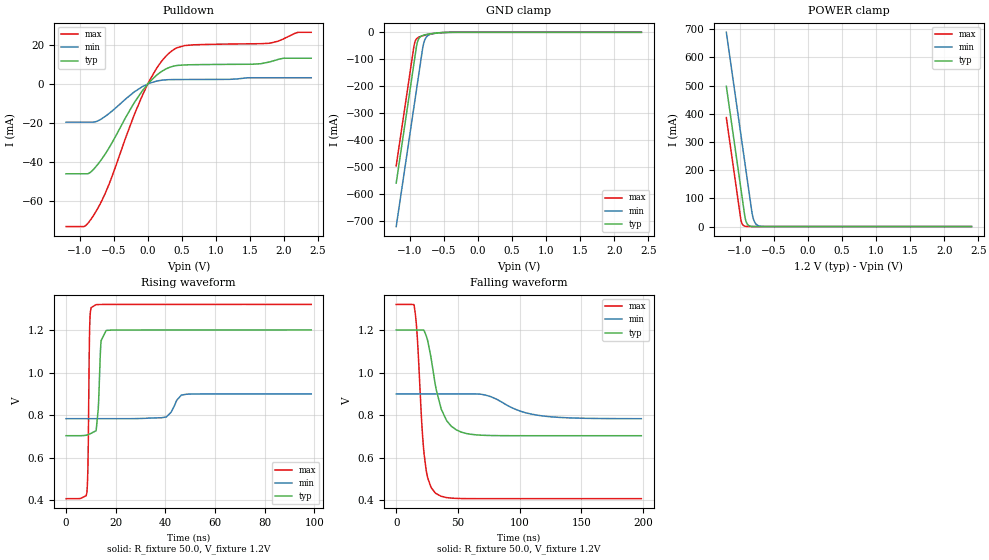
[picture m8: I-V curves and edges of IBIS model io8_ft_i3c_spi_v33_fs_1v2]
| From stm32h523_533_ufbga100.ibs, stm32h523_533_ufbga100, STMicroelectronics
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[Model]   io8_ft_i3c_spi_v33_fs_1v2
Model_type I/O_open_drain
Polarity   Non-Inverting
Enable   Active-Low
| CAP_THRESHOLD on pad IOFT is "UDTCAPC" :
| Rising=20.0% of vddiom   Falling=80.0% of vddiom
| C_comp min and max val. don't necessarily correlate with the min and max pvt
| but are the smallest and greatest pad capacitance found.
| var   typ   min   max
C_comp   3.39520pF  3.36985pF  3.42675pF
|C_comp_pulldown   3.39520pF  3.36985pF  3.42675pF
Vinl = 450.0mV
Vinh = 660.0mV
Vmeas = 600.0mV   | Reference voltage for timing measurements
Cref  = 50.0pF   | Timing specification test load capacitance value
Rref  = 1.0MOhm   | Timing specification test load resistance value
Vref  = 660.0mV   | Timing specification test load voltage
[Model Spec]
| TIME_THRESHOLD on pin ZII2CV11 is "CMOS" :
| Rising=40.0% of vdd   Falling=60.0% of vdd
Vinl 437.80000mV 335.80000mV 479.80000mV
Vinh 728.20000mV 529.20000mV 807.20000mV
| variable   typ   min   max
[Temperature Range] 25.0 125.0 -40.0
| variable   typ   min   max
[Voltage Range] 1.2V 900.0mV 1.32V
| variable   typ   min   max
[POWER Clamp Reference] 1.2V 900.0mV 1.32V
| variable   typ   min   max
[GND Clamp Reference] 0V 0V 0V
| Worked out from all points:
|   slope of the pulldown table from 0 to 0.18 V, typ, clamps not added: 30.6 ohm
|   GND clamp passes 1 mA (typ) near -0.52 V on its own axis
|   POWER clamp passes 1 mA (typ) near -0.84 V on its own axis
|   rising waveform, R_fixture 50.0, V_fixture 1.2V: 20-80 % time 1.11ns typ, 3.39ns min, 533ps max; typ from 0.704 V to 1.2 V
|   falling waveform, R_fixture 50.0, V_fixture 1.2V: 20-80 % time 11.4ns typ, 27.5ns min, 5.82ns max; typ from 1.2 V to 0.704 V
[POWER Clamp]
-1.2V     497.8mA    689.2mA    386.5mA
-990mV    140.8mA    332.2mA    29.53mA
-980mV    123.8mA    315.2mA    17.95mA
-960mV    89.81mA    281.2mA    6.634mA
-930mV    38.81mA    230.2mA    1.49mA
-900mV    12.07mA    179.2mA    334.8uA
-870mV    3.756mA    128.2mA    75.22uA
-820mV    536.4uA    44.98mA    6.246uA
-790mV    166.9uA    18.76mA    1.403uA
-750mV    35.18uA    5.846mA    191.8nA
-590mV    70.09nA    55uA       165.5pA
2.4V      0A         0A         0A
[GND Clamp]
-1.2V     -558.2mA   -719mA     -494.1mA
-940mV    -116.2mA   -277mA     -52.06mA
-930mV    -99.19mA   -260mA     -39.94mA
-900mV    -49.1mA    -209mA     -23.76mA
-880mV    -30.14mA   -175mA     -19.6mA
-850mV    -17.82mA   -124mA     -16.09mA
-810mV    -11.73mA   -56.78mA   -12.91mA
-780mV    -9.444mA   -28.21mA   -10.92mA
-740mV    -7.291mA   -13.16mA   -8.574mA
-640mV    -3.573mA   -4.171mA   -3.954mA
-380mV    -61.75uA   -230.3uA   -20.32uA
2.4V      3.863nA    718.4nA    150.6pA
| variable   typ   min   max
[Pullup Reference] 1.2V 900.0mV 1.32V
| variable   typ   min   max
[Pulldown Reference] 0V 0V 0V
[Pulldown]
-1.2V     -46.17mA   -19.62mA   -73.27mA
-930mV    -46.17mA   -19.62mA   -73.18mA
-770mV    -42.8mA    -19.41mA   -66.04mA
-570mV    -32.88mA   -15.18mA   -51.58mA
-200mV    -9.658mA   -4.083mA   -15.89mA
-80mV     -3.488mA   -1.363mA   -5.887mA
120mV     4.232mA    1.387mA    7.501mA
340mV     8.782mA    2.251mA    16.66mA
540mV     9.805mA    2.305mA    19.74mA
1.79V     11.33mA    3.206mA    20.93mA
2.2V      13.23mA    3.206mA    26.48mA
2.4V      13.23mA    3.206mA    26.56mA
[Ramp]
dV/dt_r 297.79762mV/1.02964ns 69.90051mV/3.06045ns 547.1337mV/532.05683ps
dV/dt_f 297.80511mV/10.9787ns 69.80217mV/27.29122ns 547.13933mV/5.72638ns
R_load = 50.0
| Removed startup time: 0s 0s 0s  .
| Removed end time: 98.75ns.
[Rising Waveform]
R_fixture   = 50.0
V_fixture   = 1.2V
V_fixture_min = 900.0mV
V_fixture_max = 1.32V
0s        703.7mV    783.5mV    408.1mV
8.35ns    706.4mV    783.5mV    435.3mV
8.85ns    708.5mV    783.5mV    589.5mV
9.5ns     711.7mV    783.5mV    1.21V
10.1ns    715.1mV    783.5mV    1.305V
12.1ns    727mV      783.5mV    1.319V
12.95ns   827.9mV    783.5mV    1.319V
14.1ns    1.15V      783.5mV    1.32V
16.15ns   1.198V     783.5mV    1.32V
98.75ns   1.2V       900mV      1.32V
| Removed startup time: 0s 0s 0s  .
| Removed end time: 198.75ns.
[Falling Waveform]
R_fixture   = 50.0
V_fixture   = 1.2V
V_fixture_min = 900.0mV
V_fixture_max = 1.32V
0s        1.2V       900mV      1.32V
14.5ns    1.2V       900mV      1.317V
16.85ns   1.2V       900mV      1.187V
22.65ns   1.197V     900mV      615.2mV
25.6ns    1.148V     900mV      504.3mV
32.45ns   919.4mV    900mV      431.5mV
41.5ns    769.9mV    900mV      412.7mV
56.8ns    714.2mV    900mV      408.4mV
117.7ns   703.7mV    797.4mV    408.1mV
198.8ns   703.7mV    783.7mV    408.1mV
